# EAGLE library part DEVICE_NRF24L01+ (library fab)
nRF24L01+ 2.4GHz Wireless Transceiver module
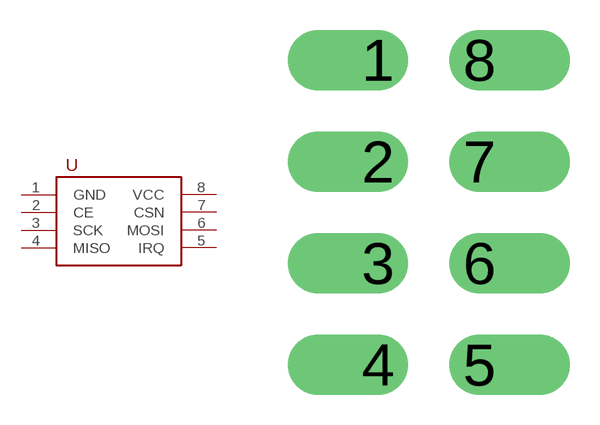
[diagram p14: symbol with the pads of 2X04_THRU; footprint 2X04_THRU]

Designator prefix -

## DEVICE_NRF24L01+  [2X04_THRU]
1  GND
2  CE
3  SCK
4  MISO
5  IRQ
6  MOSI
7  CSN
8  VCC

## Footprint 2X04_THRU (pad centres in mm)
2x4 header. Meant for nRF24L01+, but could be used for any header or 2x4 part. Extra-wide pads for greater durability in soldering.
drill 1 offset: 1 -1.27,3.81; 2 -1.27,1.27; 3 -1.27,-1.27; 4 -1.27,-3.81; 5 1.27,-3.81; 6 1.27,-1.27; 7 1.27,1.27; 8 1.27,3.81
